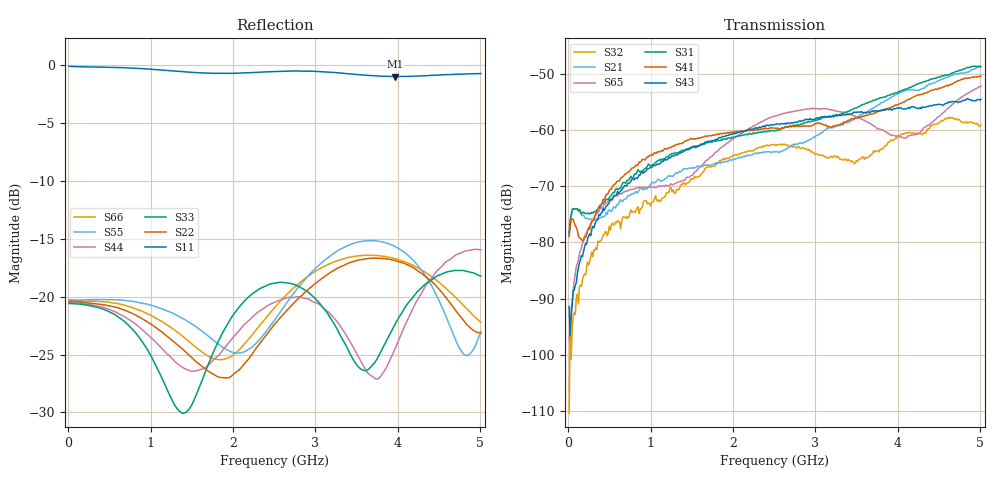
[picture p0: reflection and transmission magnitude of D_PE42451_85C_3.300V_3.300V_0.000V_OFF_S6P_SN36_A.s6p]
! Device ID: PE42451
! Serial: 36
! Insertion: A
! Temp: 85C
! VDD: 3.300
! Control_Hi: 100.000
! Control_Lo: 0.000
! Logic State: OFF
! Port 1: RFC
! Port 2: RF1
! Port 3: RF2
! Port 4: RF3
! Port 5: RF4
! Port 6: RF5
! V1 = 0.00
! V2 = 3.30
! V3 = 3.30
! V4 = 0.00
! IDD: 1.708790e-05
#  Hz  S  RI  R  50
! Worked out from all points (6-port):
!   401 points, 10 MHz to 5.01 GHz, reference 50 ohm
!   strongest paths, dB at 10 MHz, 1.26 GHz, 2.51 GHz, 3.76 GHz, 5.01 GHz:
!     S43: -91.4, -64.5, -59.0, -56.6, -54.5
!     S41: -78.9, -62.9, -59.6, -56.6, -50.3
!     S31: -78.4, -64.1, -60.1, -54.4, -48.6
!     S65: -97.3, -69.8, -57.5, -59.8, -52.2
!     S21: -78.6, -68.1, -63.9, -55.5, -48.7
!     S32: -110.4, -70.9, -62.6, -63.7, -59.1
!   lowest |S11| = -1.0 dB at 3.973 GHz (marker M1), VSWR 17.17, Z = 3.15 - j14.3 ohm
!   |S11| at or under -10 dB: nowhere
